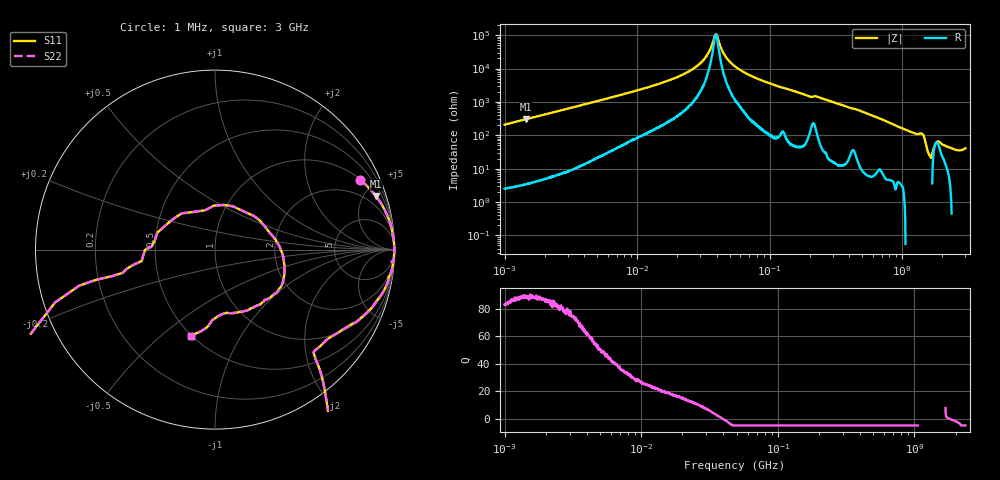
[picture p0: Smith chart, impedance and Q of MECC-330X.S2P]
!s-Parameter Generated by FASTRON Sdn. Bhd.
!FASTRON P/N : MECC-330X
!Keysight Technologies,E4991B,MY54100416,A.01.15
!Date: Thu Aug 20 11:35:05 2026
!Version  : Rev00 Thu Aug 20 11:35:05 2026
!Data & Calibration Information:
!PortZ  Port1:50+j0  Port2:50+j0
!When reading, reference impedance value at option line is always used.
!Remarks : This data is being provided solely for informational purposes.
!Freq	S11	S21	S12	S22
# Hz S dB R 50
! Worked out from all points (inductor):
!   1601 points, 1 MHz to 3 GHz, reference 50 ohm
!   read as one part in series: L = 33.1 uH near 1.041 MHz
!   highest Q = 89 at 1.448 MHz (marker M1), where L = 33.2 uH
!   self-resonance near 39.17 MHz
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1000000  -0.94 25.5  -7.32 -63.8  -7.32 -63.8  -0.94 25.5
1448161  -0.48 18.3  -10.08 -71.1  -10.08 -71.1  -0.48 18.3
3804036  -0.08 7.1  -18.14 -82.0  -18.14 -82.0  -0.08 7.1
1.447069e7  -0.02 1.7  -30.73 -85.4  -30.73 -85.4  -0.02 1.7
2.886629e7  -0.01 0.5  -41.98 -82.5  -41.98 -82.5  -0.01 0.5
3.404917e7  -0.01 0.2  -48.64 -74.4  -48.64 -74.4  -0.01 0.2
3.917023e7  -0.01 0.0  -60.41 -5.3  -60.41 -5.3  -0.01 0.0
4.597255e7  -0.01 -0.2  -47.78 77.5  -47.78 77.5  -0.01 -0.2
5.477226e7  -0.01 -0.5  -41.26 84.2  -41.26 84.2  -0.01 -0.5
2.083556e8  -0.11 -4.0  -23.10 78.1  -23.10 78.1  -0.11 -4.0
7.925923e8  -0.74 -22.2  -8.45 66.7  -8.45 66.7  -0.74 -22.2
1.287806e9  -2.02 -46.0  -2.79 51.8  -2.79 51.8  -2.02 -46.0
1.395152e9  0.11 -52.6  -1.00 64.4  -1.00 64.4  0.11 -52.6
1.430499e9  2.14 -62.4  1.62 70.2  1.62 70.2  2.14 -62.4
1.452135e9  4.08 -74.0  4.27 70.0  4.27 70.0  4.08 -74.0
1.496395e9  3.59 -140.1  7.49 24.2  7.49 24.2  3.59 -140.1
1.534307e9  -3.33 -165.7  4.45 5.8  4.45 5.8  -3.33 -165.7
1.57318e9  -7.68 -171.2  2.98 2.6  2.98 2.6  -7.68 -171.2
1.645649e9  -12.35 119.6  1.13 -10.6  1.13 -10.6  -12.35 119.6
1.818868e9  -8.25 -8.9  -4.14 5.5  -4.14 5.5  -8.25 -8.9
2.020405e9  -7.96 -43.9  -2.34 21.3  -2.34 21.3  -7.96 -43.9
3e9  -6.03 -105.5  1.81 23.0  1.81 23.0  -6.03 -105.5
